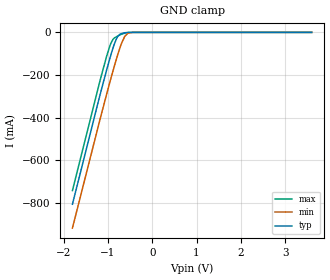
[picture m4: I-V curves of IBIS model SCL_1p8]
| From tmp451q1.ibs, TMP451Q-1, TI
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|   Model
[Model]   SCL_1p8
Model_type   Input
Vinl = .45
Vinh = 1.4
|   typ   min   max
C_comp   1.48pF   1.45pF   1.48pF
[Voltage Range]   1.8   1.7   2
[Temperature Range]   25   125   -40
[Power Clamp Reference]   1.8   1.7   2
[GND Clamp Reference]   0   0   0
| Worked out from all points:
|   GND clamp passes 1 mA (typ) near -0.57 V on its own axis
[GND Clamp]
|   Voltage   I(typ)   I(min)   I(max)
-1.8V     -807.5mA   -919.8mA   -743.4mA
-1.19V    -304mA     -418.9mA   -237.3mA
-1.033V   -180.7mA   -294.6mA   -116.1mA
-973.8mV  -135.9mA   -248.5mA   -75.23mA
-930.6mV  -104.7mA   -215.5mA   -50.48mA
-882mV    -71.9mA    -179mA     -32.07mA
-779.4mV  -20.12mA   -105.8mA   -17.46mA
-687.6mV  -5.076mA   -49.3mA    -8.576mA
-622.8mV  -2.056mA   -20.24mA   -4.029mA
-547.2mV  -480.1uA   -4.063mA   -924.5uA
-374.4mV  -2.085uA   -36.14uA   -1.054uA
3.6V      0A         0A         0A
